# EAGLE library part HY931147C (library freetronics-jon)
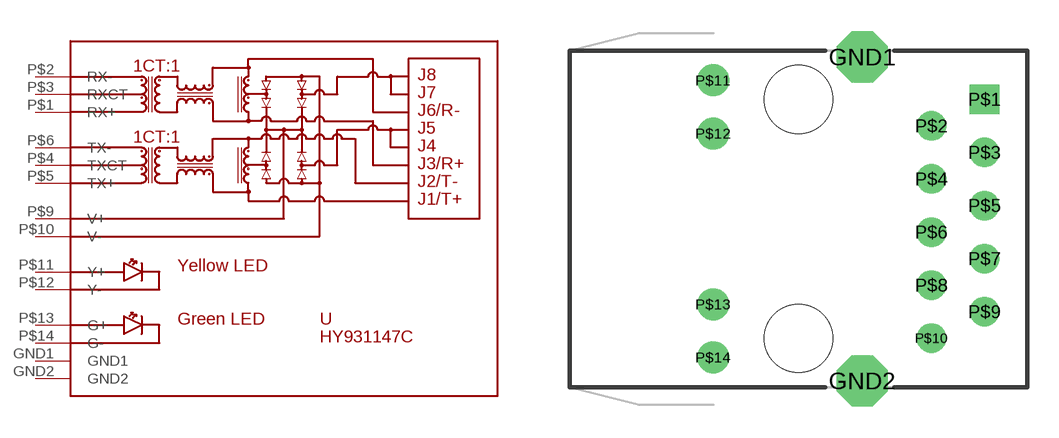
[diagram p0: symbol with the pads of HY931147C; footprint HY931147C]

Designator prefix -

## HY931147C-RJ45  [HY931147C]
GND1  GND1
GND2  GND2
P$1  RX+
P$2  RX-
P$3  RXCT
P$4  TXCT
P$5  TX+
P$6  TX-
P$9  V+
P$10  V-
P$11  Y+
P$12  Y-
P$13  G+
P$14  G-

## Footprint HY931147C (pad centres in mm)
HY931147C RJ45 Ethernet jack with built-in magnetics and PoE support
drill 1.63 octagon: GND1 3.05,7.745; GND2 3.05,-7.745
drill 0.9 square: P$1 8.89,5.715
drill 0.9: P$2 6.35,4.445; P$3 8.89,3.175; P$4 6.35,1.905; P$5 8.89,0.635; P$6 6.35,-0.635; P$7 8.89,-1.905; P$8 6.35,-3.175; P$9 8.89,-4.445; P$10 6.35,-5.715
drill 1.016: P$11 -4.08,6.625; P$12 -4.08,4.085; P$13 -4.08,-4.085; P$14 -4.08,-6.625
hole 3.25 at 0,5.715
hole 3.25 at 0,-5.715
